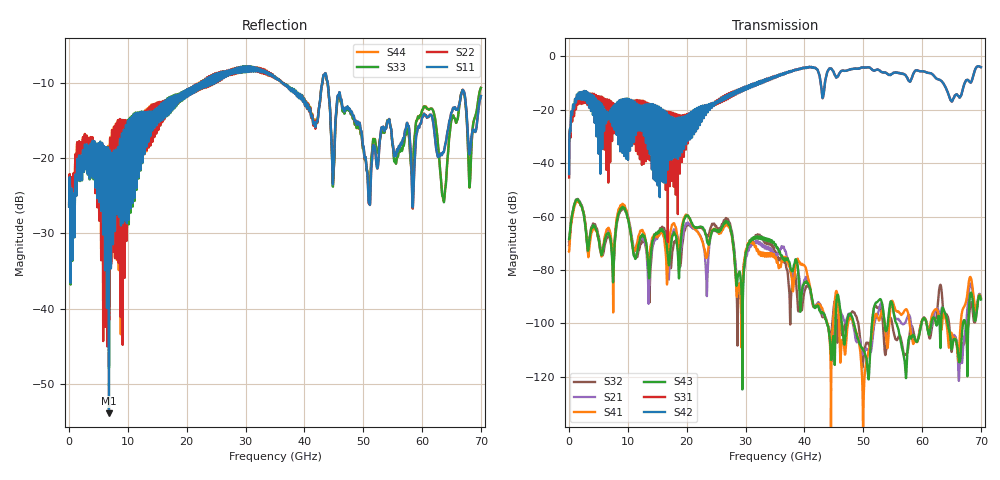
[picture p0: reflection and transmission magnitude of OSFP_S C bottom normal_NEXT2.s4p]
! AWR Design Environment (8415) Mon Jan 07 17:11:29 2019
! Document = 'OSFP Channel_S'
! nPorts: 4, nXvals: 7001
# HZ S DB R 50
!Freq DBS11 AngS11 DBS12 AngS12 DBS13 AngS13 DBS14 AngS14
!	DBS21 AngS21 DBS22 AngS22 DBS23 AngS23 DBS24 AngS24
!	DBS31 AngS31 DBS32 AngS32 DBS33 AngS33 DBS34 AngS34
!	DBS41 AngS41 DBS42 AngS42 DBS43 AngS43 DBS44 AngS44
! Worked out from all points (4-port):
!   7000 points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, 10 MHz to 70 GHz, reference 50 ohm
!   strongest paths, dB at 10 MHz, 17.51 GHz, 35.01 GHz, 52.51 GHz, 70 GHz:
!     S42: -44.0, -28.3, -7.4, -4.9, -4.0
!     S31: -45.4, -27.5, -7.4, -4.9, -4.0
!     S43: -68.5, -67.5, -70.6, -91.7, -91.0
!     S41: -73.1, -63.0, -75.6, -97.9, -90.5
!     S21: -70.8, -66.7, -74.5, -96.2, -90.3
!     S32: -69.5, -73.8, -73.1, -94.2, -90.8
!   lowest |S11| = -53.9 dB at 6.78 GHz (marker M1), VSWR 1.00, Z = 50.1 - j0.161 ohm
!   |S11| at or under -10 dB: start of sweep to 22.43 GHz; 36.26 GHz to 43.05 GHz (6.791 GHz wide, 17.1 % of centre); 43.96 GHz to end of sweep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
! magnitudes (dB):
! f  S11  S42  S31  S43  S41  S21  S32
! 10 MHz  -26.5  -44.0  -45.4  -68.5  -73.1  -70.8  -69.5
! 1.62 GHz  -21.3  -13.5  -15.0  -54.2  -54.6  -54.3  -54.0
! 3.3 GHz  -18.7  -14.7  -14.2  -71.8  -75.1  -73.3  -71.9
! 6.78 GHz  -53.9  -22.2  -17.1  -66.4  -64.5  -65.6  -67.4
! 30.88 GHz  -7.8  -10.5  -10.6  -69.3  -69.7  -71.3  -70.0
! 63.65 GHz  -19.2  -10.2  -10.2  -94.7  -96.4  -95.2  -96.6
! 70 GHz  -11.8  -4.0  -4.0  -91.0  -90.5  -90.3  -90.8
